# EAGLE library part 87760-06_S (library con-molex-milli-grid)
HEADER
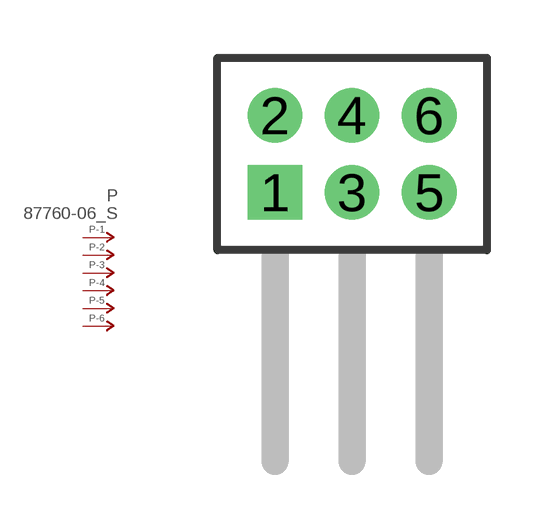
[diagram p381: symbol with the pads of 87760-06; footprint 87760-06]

Designator prefix P; gates -1=P-NV -2=P-N -3=P-N -4=P-N -5=P-N -6=P-N

## 87760-06_S  [87760-06]
1  -1:P  pas
2  -2:P  pas
3  -3:P  pas
4  -4:P  pas
5  -5:P  pas
6  -6:P  pas

## Footprint 87760-06 (pad centres in mm)
HEADER Dual Row, Right Angle
drill 0.914 square: 1 -2,-1
drill 0.914: 2 -2,1; 3 0,-1; 4 0,1; 5 2,-1; 6 2,1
